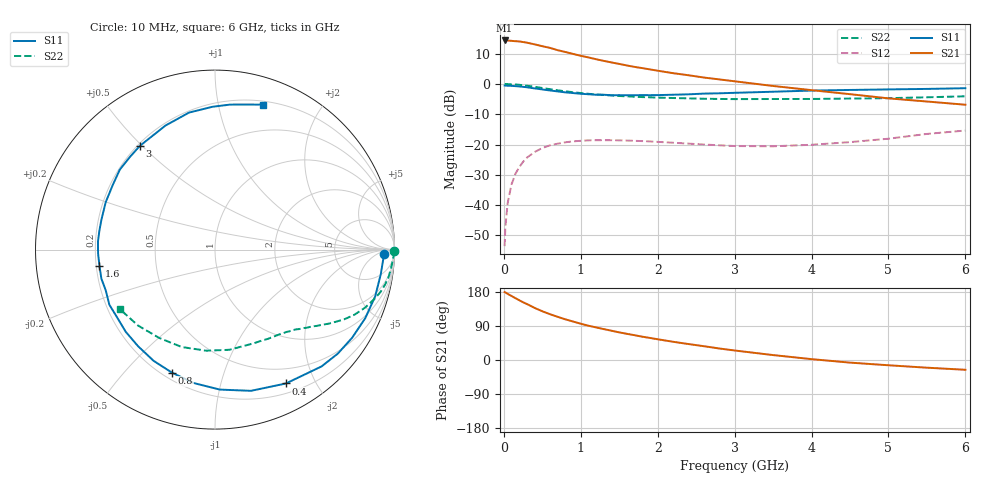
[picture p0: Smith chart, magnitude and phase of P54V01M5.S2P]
! SIEMENS Small Signal Semiconductors
! BFP183
! Si NPN RF Bipolar Junction Transistor in SOT143
! VCE = 4 V  IC = 1.5 mA
! Common Emitter S-Parameters:  March  1996
# GHz  S  MA  R  50
!  f  S11  S21  S12  S22
! GHz  MAG  ANG  MAG  ANG  MAG  ANG  MAG  ANG
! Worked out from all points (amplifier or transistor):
!   36 points, 10 MHz to 6 GHz, reference 50 ohm
!   highest |S21| = 14.4 dB at 10 MHz (marker M1)
!   |S21| within 3 dB of that: start of sweep to 672 MHz
!   unconditionally stable (mu >= 1): 2.284 GHz to 5.896 GHz
!   at 250 MHz: K = 0.11, MSG = 19.8 dB, |S12| = -25.7 dB
!   at 1.4 GHz: K = 0.60, MSG = 12.8 dB, |S12| = -18.6 dB
!   at 6 GHz: K = 0.97, MSG = 4.3 dB, |S12| = -15.4 dB
!   S11 on the Smith chart (normalised r, x): 10 MHz: 29, -12; 400 MHz: 0.31, -1.62; 800 MHz: 0.24, -0.68; 1.6 GHz: 0.21, -0.07; 3 GHz: 0.21, +0.49; 6 GHz: 0.23, +1.36
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0.01  0.9415 -1.4  5.222 179.2  0.0021 87.5  1 -0.6
0.02  0.939 -3.2  5.188 178.3  0.0044 84.5  0.9985 -1.3
0.05  0.9338 -8.4  5.202 174.4  0.0109 87.6  0.9935 -2.9
0.1  0.9298 -16.2  5.146 168.9  0.022 79.5  0.9864 -5.9
0.2  0.9083 -32.7  5.031 157.7  0.0424 71.5  0.9675 -11.6
0.25  0.8968 -40.2  4.919 152.3  0.0518 66.7  0.9522 -14.3
0.4  0.8441 -62.1  4.503 137.5  0.0753 54.9  0.8971 -21.1
0.5  0.812 -75.7  4.197 128.6  0.0875 47.7  0.8579 -25.0
0.6  0.7804 -88.0  3.939 120.9  0.097 41.6  0.8198 -28.2
0.7  0.7527 -99.1  3.607 113.9  0.1033 36.3  0.7849 -30.8
0.8  0.7264 -109.2  3.366 107.3  0.1088 31.7  0.7557 -33.1
1  0.688 -128.6  2.915 95.7  0.1151 23.8  0.7079 -36.9
1.1  0.676 -137.4  2.74 90.4  0.1172 20.8  0.6872 -38.6
1.3  0.6638 -152.5  2.401 81.5  0.1179 15.2  0.6567 -41.8
1.6  0.6501 -172.0  2.018 69.1  0.1163 9.5  0.6244 -46.0
1.8  0.6536 176.1  1.826 61.5  0.1139 7.0  0.6069 -49.1
2.2  0.6637 156.6  1.506 48.1  0.1071 3.5  0.5856 -55.6
3  0.7136 126.0  1.106 25.1  0.0944 5.9  0.5615 -71.0
3.5  0.7441 111.8  0.926 13.0  0.0935 11.7  0.5639 -81.9
4.5  0.7959 91.0  0.678 -6.9  0.1096 22.8  0.5735 -108.9
5.5  0.8279 77.5  0.513 -20.3  0.1496 25.5  0.6024 -135.4
6  0.8502 71.8  0.454 -25.8  0.1703 22.3  0.6258 -148.1
